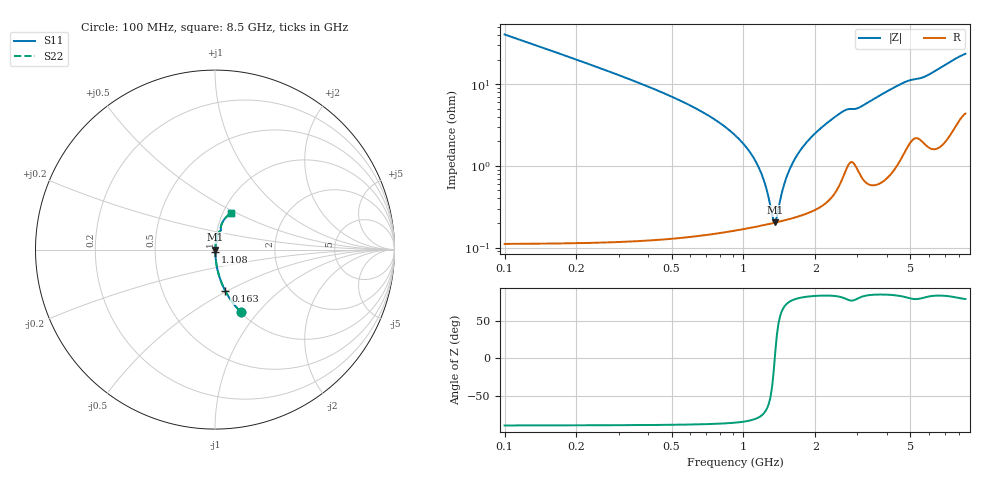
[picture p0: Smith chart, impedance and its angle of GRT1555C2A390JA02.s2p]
!Murata Part Number: GRT1555C2A390JA02
!These Parameters are Measured in Series Mode Connection
!Data Generated on Jun 19, 2026
!  o--ll--o
!Port1  Port2
!  o------o
!Operation Temp=25[degC], DC Bias Voltage=0[V]
!Freq. Start=100[MHz] Stop=9[GHz] 401[Steps]
# Hz S RI R 50
!Freq.(Hz) S11(Real) S11(Imag) S21(Real) S21(Imag) S12(Real) S12(Imag) S22(Real) S22(Imag)
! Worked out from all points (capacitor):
!   401 points, 100 MHz to 8.5 GHz, reference 50 ohm
!   read as one part in series: C = 39 pF near 142 MHz
!   lowest |Z| = 205 mohm at 1.36 GHz (marker M1)
!   series resonance near 1.353 GHz, so ESL is about 350 pH
!   S11 on the Smith chart (normalised r, x): 100 MHz: 1.00, -0.81; 163 MHz: 1.00, -0.49; 1.108 GHz: 1.00, -0.02; 8.5 GHz: 1.09, +0.46
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1e8  0.1421 -0.3478  0.8579 0.3478  0.8579 0.3478  0.1421 -0.3478
1.63e8  0.0583 -0.2321  0.9417 0.2321  0.9417 0.2321  0.0583 -0.2321
2.47e8  0.0259 -0.1554  0.9741 0.1554  0.9741 0.1554  0.0259 -0.1554
3.73e8  0.0113 -0.0998  0.9887 0.0998  0.9887 0.0998  0.0113 -0.0998
8.98e8  0.00223 -0.0253  0.9978 0.0253  0.9978 0.0253  0.00223 -0.0253
1.108e9  0.00192 -0.0121  0.9981 0.0121  0.9981 0.0121  0.00192 -0.0121
1.213e9  0.00192 -0.0066  0.9981 0.0066  0.9981 0.0066  0.00192 -0.0066
1.318e9  0.00198 -0.00157  0.998 0.00157  0.998 0.00157  0.00198 -0.00157
1.36e9  0.00202 0.000325  0.998 -0.000325  0.998 -0.000325  0.00202 0.000325
1.381e9  0.00204 0.00125  0.998 -0.00125  0.998 -0.00125  0.00204 0.00125
1.465e9  0.00215 0.00484  0.9979 -0.00484  0.9979 -0.00484  0.00215 0.00484
1.507e9  0.00221 0.00657  0.9978 -0.00657  0.9978 -0.00657  0.00221 0.00657
1.591e9  0.00236 0.00992  0.9976 -0.00992  0.9976 -0.00992  0.00236 0.00992
1.696e9  0.00259 0.0139  0.9974 -0.0139  0.9974 -0.0139  0.00259 0.0139
1.99e9  0.00347 0.0245  0.9965 -0.0245  0.9965 -0.0245  0.00347 0.0245
2.557e9  0.00816 0.0436  0.9918 -0.0436  0.9918 -0.0436  0.00816 0.0436
2.914e9  0.0127 0.0474  0.9873 -0.0474  0.9873 -0.0474  0.0127 0.0474
4.3e9  0.0171 0.0891  0.9829 -0.0891  0.9829 -0.0891  0.0171 0.0891
4.867e9  0.0277 0.1032  0.9723 -0.1032  0.9723 -0.1032  0.0277 0.1032
5.707e9  0.0321 0.1152  0.9679 -0.1152  0.9679 -0.1152  0.0321 0.1152
7.114e9  0.0489 0.1645  0.9511 -0.1645  0.9511 -0.1645  0.0489 0.1645
8.5e9  0.0867 0.2023  0.9133 -0.2023  0.9133 -0.2023  0.0867 0.2023
